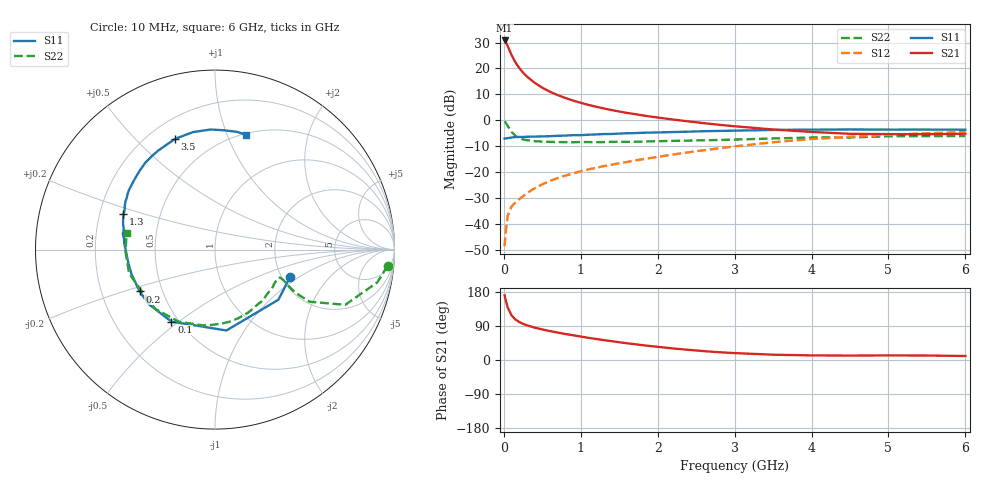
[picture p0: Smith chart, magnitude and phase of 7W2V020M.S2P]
! Infineon Technologies  Discrete & RF Semiconductors
! BFS17W
! Si NPN RF Bipolar Junction Transistor in SOT323
! VCE = 2 V  IC = 20 mA
! Common Emitter S-Parameters:  August  1999
# GHz  S  MA  R  50
!  f  S11  S21  S12  S22
! GHz  MAG  ANG  MAG  ANG  MAG  ANG  MAG  ANG
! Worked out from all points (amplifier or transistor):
!   36 points, 10 MHz to 6 GHz, reference 50 ohm
!   highest |S21| = 30.8 dB at 10 MHz (marker M1)
!   |S21| within 3 dB of that: start of sweep to 62.67 MHz
!   unconditionally stable (mu >= 1): 234.1 MHz to 2.786 GHz; 4.034 GHz to end of sweep
!   at 250 MHz: K = 1.04, MAG = 22.6 dB, |S12| = -29.2 dB
!   at 1.4 GHz: K = 1.24, MAG = 7.6 dB, |S12| = -17.1 dB
!   at 6 GHz: K = 1.09, MAG = -2.2 dB, |S12| = -4.4 dB
!   S11 on the Smith chart (normalised r, x): 10 MHz: 2.23, -0.83; 100 MHz: 0.46, -0.47; 200 MHz: 0.37, -0.22; 1.3 GHz: 0.30, +0.17; 3.5 GHz: 0.30, +0.66; 6 GHz: 0.51, +1.17
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0.01  0.4454 -19.7  34.62 170.7  0.0038 82.7  0.9655 -5.4
0.02  0.4503 -38.3  33.38 161.1  0.0062 81.5  0.9226 -11.4
0.05  0.4552 -82.0  27.12 138.7  0.0147 64.6  0.7878 -23.0
0.1  0.4687 -121.2  18.18 118.0  0.022 56.1  0.6002 -28.9
0.15  0.4783 -140.6  13.18 107.0  0.0264 56.5  0.5043 -28.1
0.2  0.4803 -151.0  10.24 100.3  0.0306 59.9  0.4587 -26.4
0.25  0.4801 -158.4  8.319 95.4  0.0347 60.1  0.4312 -24.9
0.3  0.4848 -163.4  6.995 91.6  0.04 62.4  0.4166 -24.0
0.4  0.4885 -170.8  5.307 85.4  0.0493 64.9  0.3981 -23.3
0.5  0.4923 -176.0  4.269 80.6  0.0589 66.8  0.3916 -23.6
0.6  0.4979 -180.0  3.563 76.3  0.0684 67.6  0.3869 -24.7
0.7  0.5064 176.5  3.077 72.4  0.0777 68.2  0.3837 -26.3
0.9  0.5209 170.4  2.409 65.2  0.0951 68.9  0.3808 -30.7
1.1  0.5312 164.5  1.992 58.4  0.1144 68.8  0.3828 -36.0
1.3  0.5468 158.8  1.7 52.4  0.1318 68.9  0.3827 -42.1
1.6  0.5666 151.8  1.397 44.2  0.1586 69.0  0.3867 -51.4
2.2  0.5974 137.9  1.04 30.5  0.221 67.7  0.4041 -71.7
2.8  0.6279 124.4  0.824 20.5  0.2912 63.8  0.4204 -92.7
3.5  0.6561 109.8  0.669 14.0  0.3804 56.9  0.4495 -116.8
4.5  0.6696 92.1  0.553 11.7  0.4833 43.6  0.4696 -151.0
5.5  0.6672 79.4  0.543 11.8  0.5662 31.4  0.4985 -178.6
6  0.6628 74.7  0.555 10.6  0.5999 25.6  0.5014 169.2
